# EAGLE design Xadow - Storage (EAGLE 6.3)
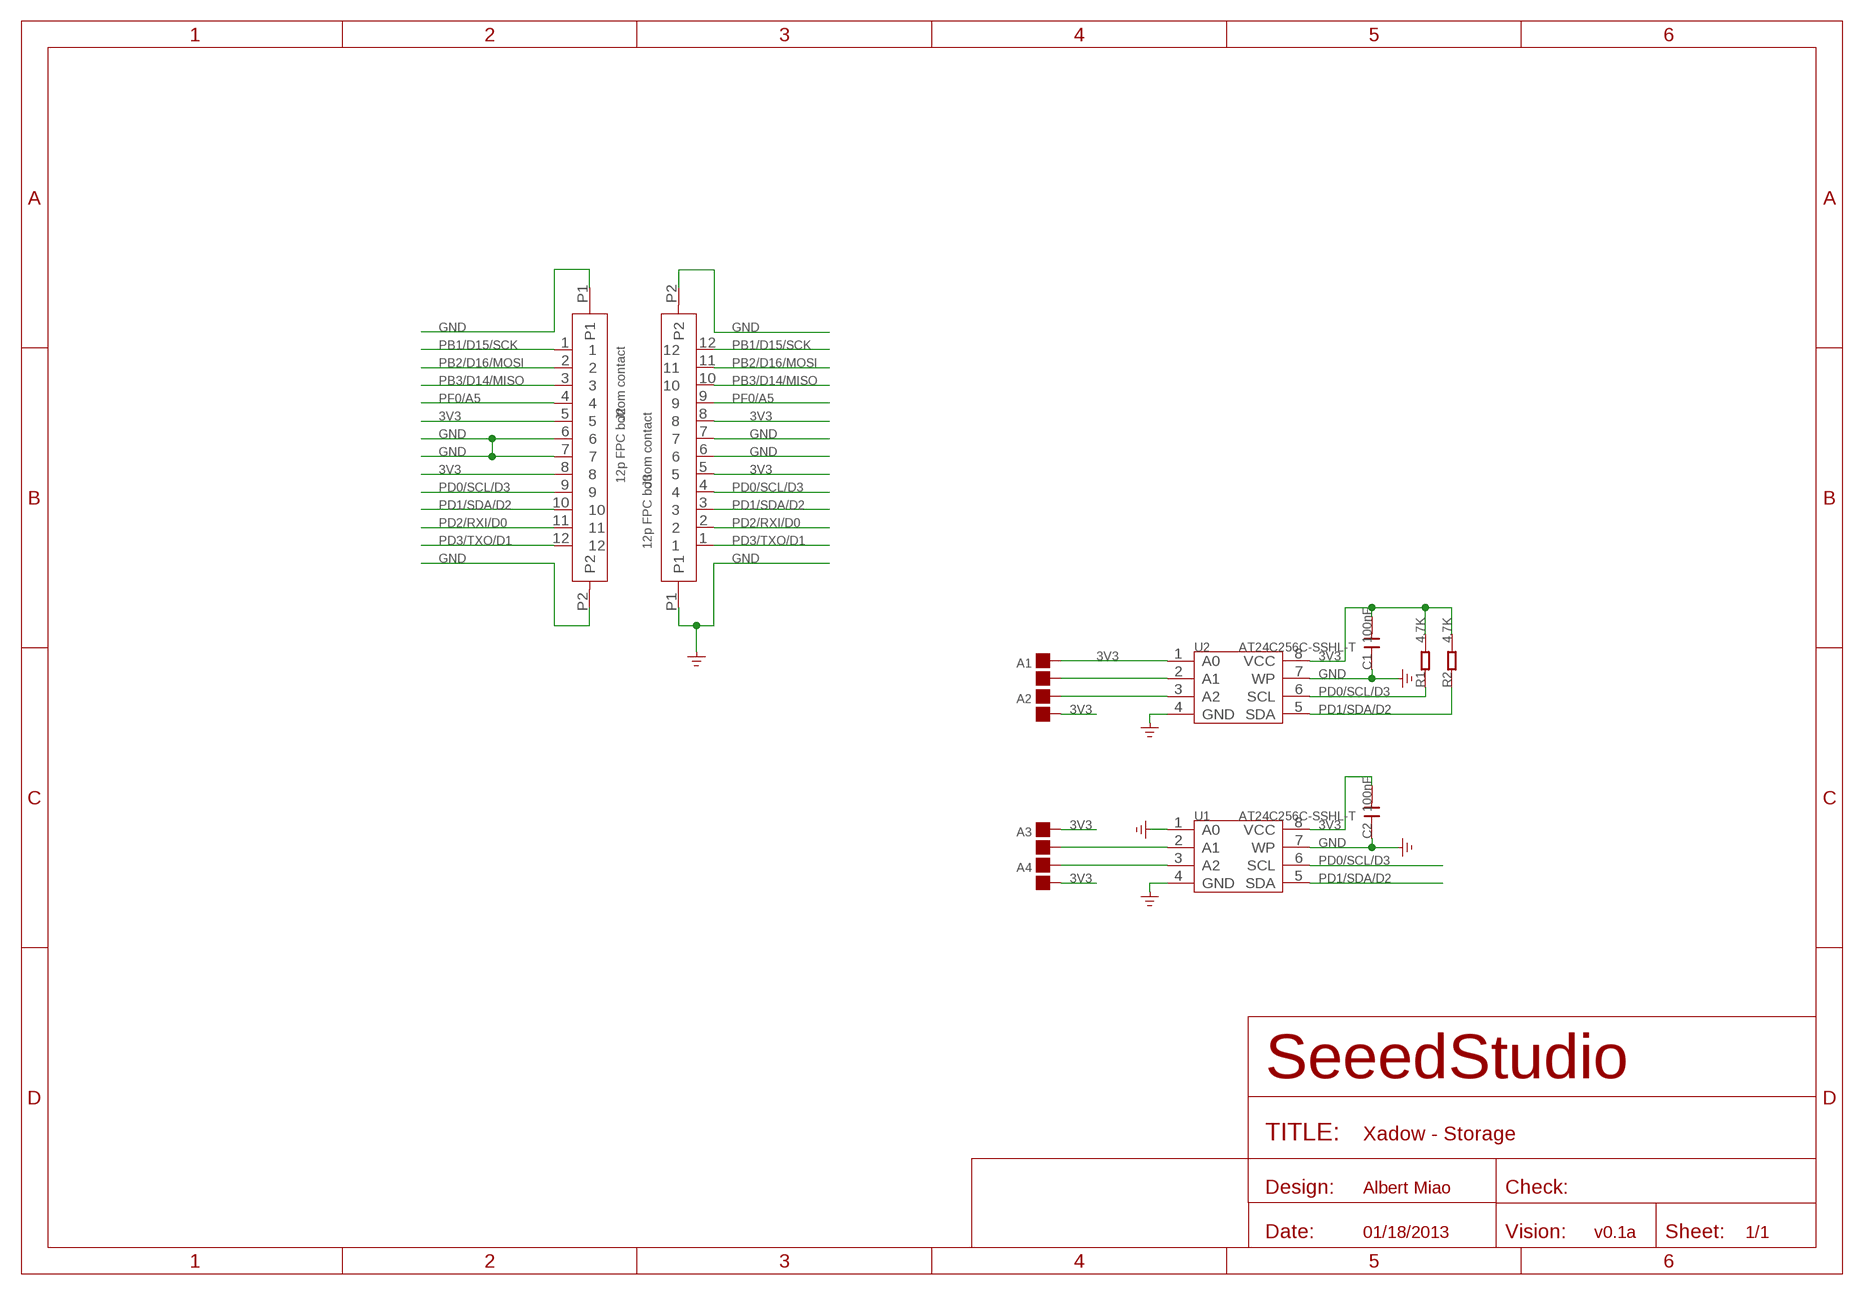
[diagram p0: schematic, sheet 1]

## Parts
A1  PAD-JUMPER-2P  [2P-SMD-1.78X1.27]
A2  PAD-JUMPER-2P  [2P-SMD-1.78X1.27]
A3  PAD-JUMPER-2P  [2P-SMD-1.78X1.27]
A4  PAD-JUMPER-2P  [2P-SMD-1.78X1.27]
C1  100nF  C-0603  [C0603]
C2  100nF  C-0603  [C0603]
J2  12p FPC bottom contact  FPC052002-12LT  [12P-0.5]
J3  12p FPC bottom contact  FPC052002-12LT  [12P-0.5]
R1  4.7K  R-0603  [R0603]
R2  4.7K  R-0603  [R0603]
U1  AT24C256C-SSHL-T  AT24C256C'  [SOIC8-6.0]
U2  AT24C256C-SSHL-T  AT24C256C'  [SOIC8-6.0]

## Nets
3V3: A1.2 A2.1 A3.2 A4.1 C1.2 C2.2 J2.5 J2.8 J3.5 J3.8 R1.2 R2.2 U1.8(VCC) U2.1(A0) U2.8(VCC)
GND: C1.1 C2.1 J2.6 J2.7 J2.P1 J2.P2 J3.6 J3.7 J3.P1 J3.P2 U1.1(A0) U1.4(GND) U1.7(WP) U2.4(GND) U2.7(WP)
N$1: A1.1 U2.2(A1)
N$2: A2.2 U2.3(A2)
N$3: A3.1 U1.2(A1)
N$4: A4.2 U1.3(A2)
PB1/D15/SCK: J2.1 J3.12
PB2/D16/MOSI: J2.2 J3.11
PB3/D14/MISO: J2.3 J3.10
PD0/SCL/D3: J2.9 J3.4 R1.1 U1.6(SCL) U2.6(SCL)
PD1/SDA/D2: J2.10 J3.3 R2.1 U1.5(SDA) U2.5(SDA)
PD2/RXI/D0: J2.11 J3.2
PD3/TXO/D1: J2.12 J3.1
PF0/A5: J2.4 J3.9

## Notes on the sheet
- Albert Miao
- 01/18/2013 | v0.1a

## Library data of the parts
A1-A4 = Discrete (1):PAD-JUMPER-2P; PARTNO: DNP
C1 C2 = Discrete (1):C*: Ceramic Capacitors
J2 J3 = template:FPC052002-12LT
R1 R2 = Discrete (1):R*
U1 U2 = template:AT24C256C: Two-wire Serial EEPROM 256K (32,768 x 8)

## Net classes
0 default: width 0.152 mm, drill 0.305 mm, clearance 0.152 mm
1 GND: width 0.152 mm, drill 0.305 mm, clearance 0.152 mm to class 0, clearance 0.152 mm
3 usbvcc: width 0.203 mm, drill 0.305 mm, clearance 0.203 mm

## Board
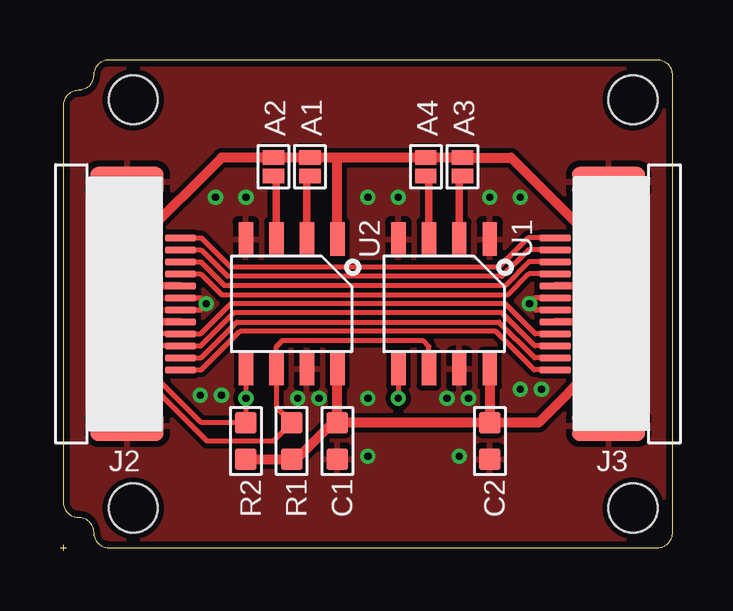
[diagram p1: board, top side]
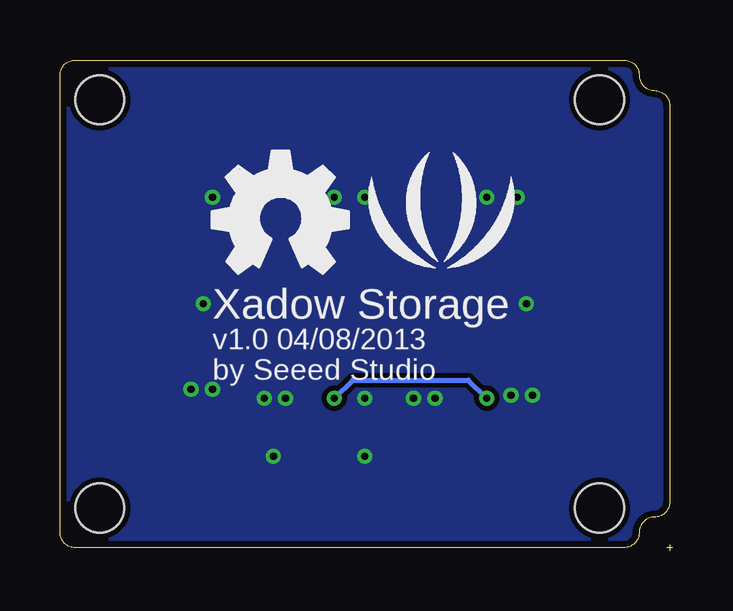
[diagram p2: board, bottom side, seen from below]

Size 25.53 x 20.45 mm. Coordinates in mm from the lower left corner, seen from the top.
Outline: 25.53,19.81 arc90 24.89,20.45
Outline: 2.03,20.45 arc90 1.4,19.81
Outline: 1.4,19.81 arc-90 0.76,19.18
Outline: 0.76,19.18 arc90 0.13,18.54
Outline: 0.13,2.03 arc90 0.76,1.4
Outline: 0.76,1.4 arc-90 1.4,0.76
Outline: 1.4,0.76 arc90 2.03,0.13
Outline: 24.89,0.13 arc90 25.53,0.76
Outline: 25.53,0.76 25.53,19.81
Outline: 25.53,19.81 arc90 24.89,20.45
Outline: 24.89,20.45 2.03,20.45
Outline: 2.03,20.45 arc90 1.4,19.81
Outline: 1.4,19.81 arc-90 0.76,19.18
Outline: 0.76,19.18 arc90 0.13,18.54
Outline: 0.13,18.54 0.13,2.03
Outline: 0.13,2.03 arc90 0.76,1.4
Outline: 0.76,1.4 arc-90 1.4,0.76
Outline: 1.4,0.76 1.4,0.76
Outline: 1.4,0.76 arc90 2.03,0.13
Outline: 2.03,0.13 24.89,0.13
Outline: 24.89,0.13 arc90 25.53,0.76
Outline: 0,0.13 0.25,0.13
Outline: 0.13,0.25 0.13,0
Copper layers (1*16): Top 0.035mm / dielectric 1.5mm / Bottom 0.035mm
Design rules "SeeedStudio_rule_no_angle_090911 *": minimum track width 6mil, minimum drill 12mil, track to track 6mil, track to pad 6mil, pad to pad 6mil, via to via 6mil, smd to smd 0mil, copper to edge 10mil, drill to drill 10mil, minimum pad ring 10mil, minimum via ring 6mil, stop-mask expansion 2mil, vias tented up to drill 25mil, thermal gap 10mil
Holes 2.03 mm at 3.05,1.78 3.05,18.8 23.88,18.8 23.88,1.78
tRestrict: area 20.3,10 to 21,10.5; area 4.8,10 to 5.3,10.5

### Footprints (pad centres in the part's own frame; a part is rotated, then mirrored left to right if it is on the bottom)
2P-SMD-1.78X1.27 = smd 0.889 x 0.61: 1 0,0.381; 2 0,-0.381
C0603 = smd 0.889 x 0.889: 1 -0.762,0; 2 0.762,0
12P-0.5 = smd 0.3 x 1.3: 1 -2.75,2.35; 2 -2.25,2.35; 3 -1.75,2.35; 4 -1.25,2.35; 5 -0.75,2.35; 6 -0.25,2.35; 7 0.25,2.35; 8 0.75,2.35; 9 1.25,2.35; 10 1.75,2.35; 11 2.25,2.35; 12 2.75,2.35 | smd 1.27 x 3.048: P1 -5.08,0.127; P2 5.08,0.127
R0603 = smd 0.889 x 0.889: 1 -0.762,0; 2 0.762,0
SOIC8-6.0 = smd 0.6 x 1.4: 1 -1.905,-2.7; 2 -0.635,-2.7; 3 0.635,-2.7; 4 1.905,-2.7; 5 1.905,2.7; 6 0.635,2.7; 7 -0.635,2.7; 8 -1.905,2.7

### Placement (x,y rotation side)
A1  10.41,16 180 top
A2  8.89,16 0 top
A3  16.76,16 180 top
A4  15.24,16 0 top
C1  11.56,4.57 90 top
C2  17.91,4.57 90 top
J2  2.67,10.29 270 top
J3  22.99,10.29 90 top
R1  9.65,4.57 270 top
R2  7.75,4.57 270 top
U1  16,10.29 180 top
U2  9.65,10.29 180 top
U$2  [LOGO_SILK]  9.65,13.46 0 bottom
U$3  [OSHW_FILLX200_NOTEXT]  19.18,11.56 0 bottom

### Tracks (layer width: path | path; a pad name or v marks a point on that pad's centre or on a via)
3V3
  Top 0.305: J2.8 4.05,9.54 3.3,10.29 | J2.5 3.57,11.04 | 3.54,11.04 3.44,11.04 3.3,11.18 | 3.57,11.04 3.3,11.3 | 3.57,11.04 3.54,11.04 | 3.54,11.04 3.3,10.8 | J3.8 21.9,11.04 22.09,11.04 | 22.09,11.04 22.34,11.04 22.35,11.05 | J3.5 22.09,9.54 | 22.11,9.54 22.34,9.54 22.35,9.53 | 22.09,9.54 22.11,9.54 | 22.11,9.54 22.35,9.78 | 22.09,9.54 22.35,9.27 | 22.09,11.04 22.35,11.3 | 22.09,11.04 22.11,11.04 22.35,10.8
  Top 0.406: 11.56,16.38 A4.1 A3.2 18.8,16.38 22.35,12.83 22.35,11.3 22.35,11.05 22.35,10.8 22.35,9.78 22.35,9.53 22.35,9.27 22.35,7.75 19.94,5.33 C2.2 | 11.56,16.38 A1.2 A2.1 6.73,16.38 3.3,12.95 3.3,11.3 3.3,11.18 3.3,10.8 3.3,10.29 | U2.1 11.56,16.38 | C1.2 U2.8 | U1.8 C2.2 | R2.2 R1.2 9.84,3.81 11.37,5.33 C1.2 | C2.2 C1.2
GND  (via drill 0.3 pad 0.64)
  Top 0.203: J3.7 19.81,10.54 v19.56,10.29 19.81,10.04 J3.6 | J2.6 5.85,10.54 v6.1,10.29 5.85,10.04 J2.7
  other vias: 17.02,6.35 19.18,6.73 20.07,6.73 6.48,14.73 7.75,14.73 14.1,14.73 12.83,14.73 17.91,14.73 19.18,14.73 9.91,6.35 10.79,6.35 16.13,6.35 5.84,6.48 6.73,6.48 12.83,6.35 12.83,3.94 16.64,3.94
  pour Top (isolate 0.203): 0.13,0.13 25.53,0.13 25.53,20.45 0.13,20.45
  pour Bottom (isolate 0.203): 0.13,0.13 25.53,0.13 25.53,20.45 0.13,20.45
N$1
  Top 0.305: U2.2 10.29,15.49 A1.1
N$2
  Top 0.305: U2.3 9.02,15.49 A2.2
N$3
  Top 0.305: U1.2 16.64,15.49 A3.1
N$4
  Top 0.305: U1.3 15.37,15.49 A4.2
PB1/D15/SCK
  Top 0.203: J3.12 19.51,13.04 18.29,11.81 7.11,11.81 5.89,13.04 J2.1
PB2/D16/MOSI
  Top 0.203: J2.2 5.88,12.54 6.99,11.43 18.41,11.43 19.52,12.54 J3.11
PB3/D14/MISO
  Top 0.203: J3.10 19.53,12.04 18.54,11.05 6.86,11.05 5.87,12.04 J2.3
PD0/SCL/D3
  Top 0.203: U1.6 15.37,8.51 15.11,8.76 9.27,8.76 9.02,8.51 U2.6 9.02,5.97 R1.1 8.89,4.57 6.13,4.57 3.43,7.27 3.43,8.38 4.08,9.04 J2.9 5.86,9.04 7.11,10.29 18.54,10.29 19.79,9.04 J3.4
PD1/SDA/D2  (via drill 0.3 pad 0.64)
  Top 0.203: U2.5 7.75,7.11 | 7.75,7.11 v7.75,6.35 7.75,5.46 7.62,5.33 | 7.62,5.33 R2.1 | J3.3 19.78,8.54 18.41,9.91 7.24,9.91 5.87,8.54 J2.10 4.09,8.54 3.81,8.26 3.81,7.42 5.89,5.33 7.62,5.33 | 7.62,6.99 7.75,7.11 | U1.5 v14.1,6.35
  Bottom 0.203: v14.1,6.35 13.34,7.11 8.51,7.11 v7.75,6.35
PD2/RXI/D0
  Top 0.203: J3.2 19.78,8.04 18.29,9.53 7.37,9.53 5.88,8.04 J2.11
PD3/TXO/D1
  Top 0.203: J3.1 19.77,7.54 18.16,9.14 7.49,9.14 5.89,7.54 J2.12
PF0/A5
  Top 0.203: J2.4 5.86,11.54 6.73,10.67 18.67,10.67 19.54,11.54 J3.9

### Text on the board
bPlace: Xadow Storage | v1.0 04/08/2013 | by Seeed Studio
